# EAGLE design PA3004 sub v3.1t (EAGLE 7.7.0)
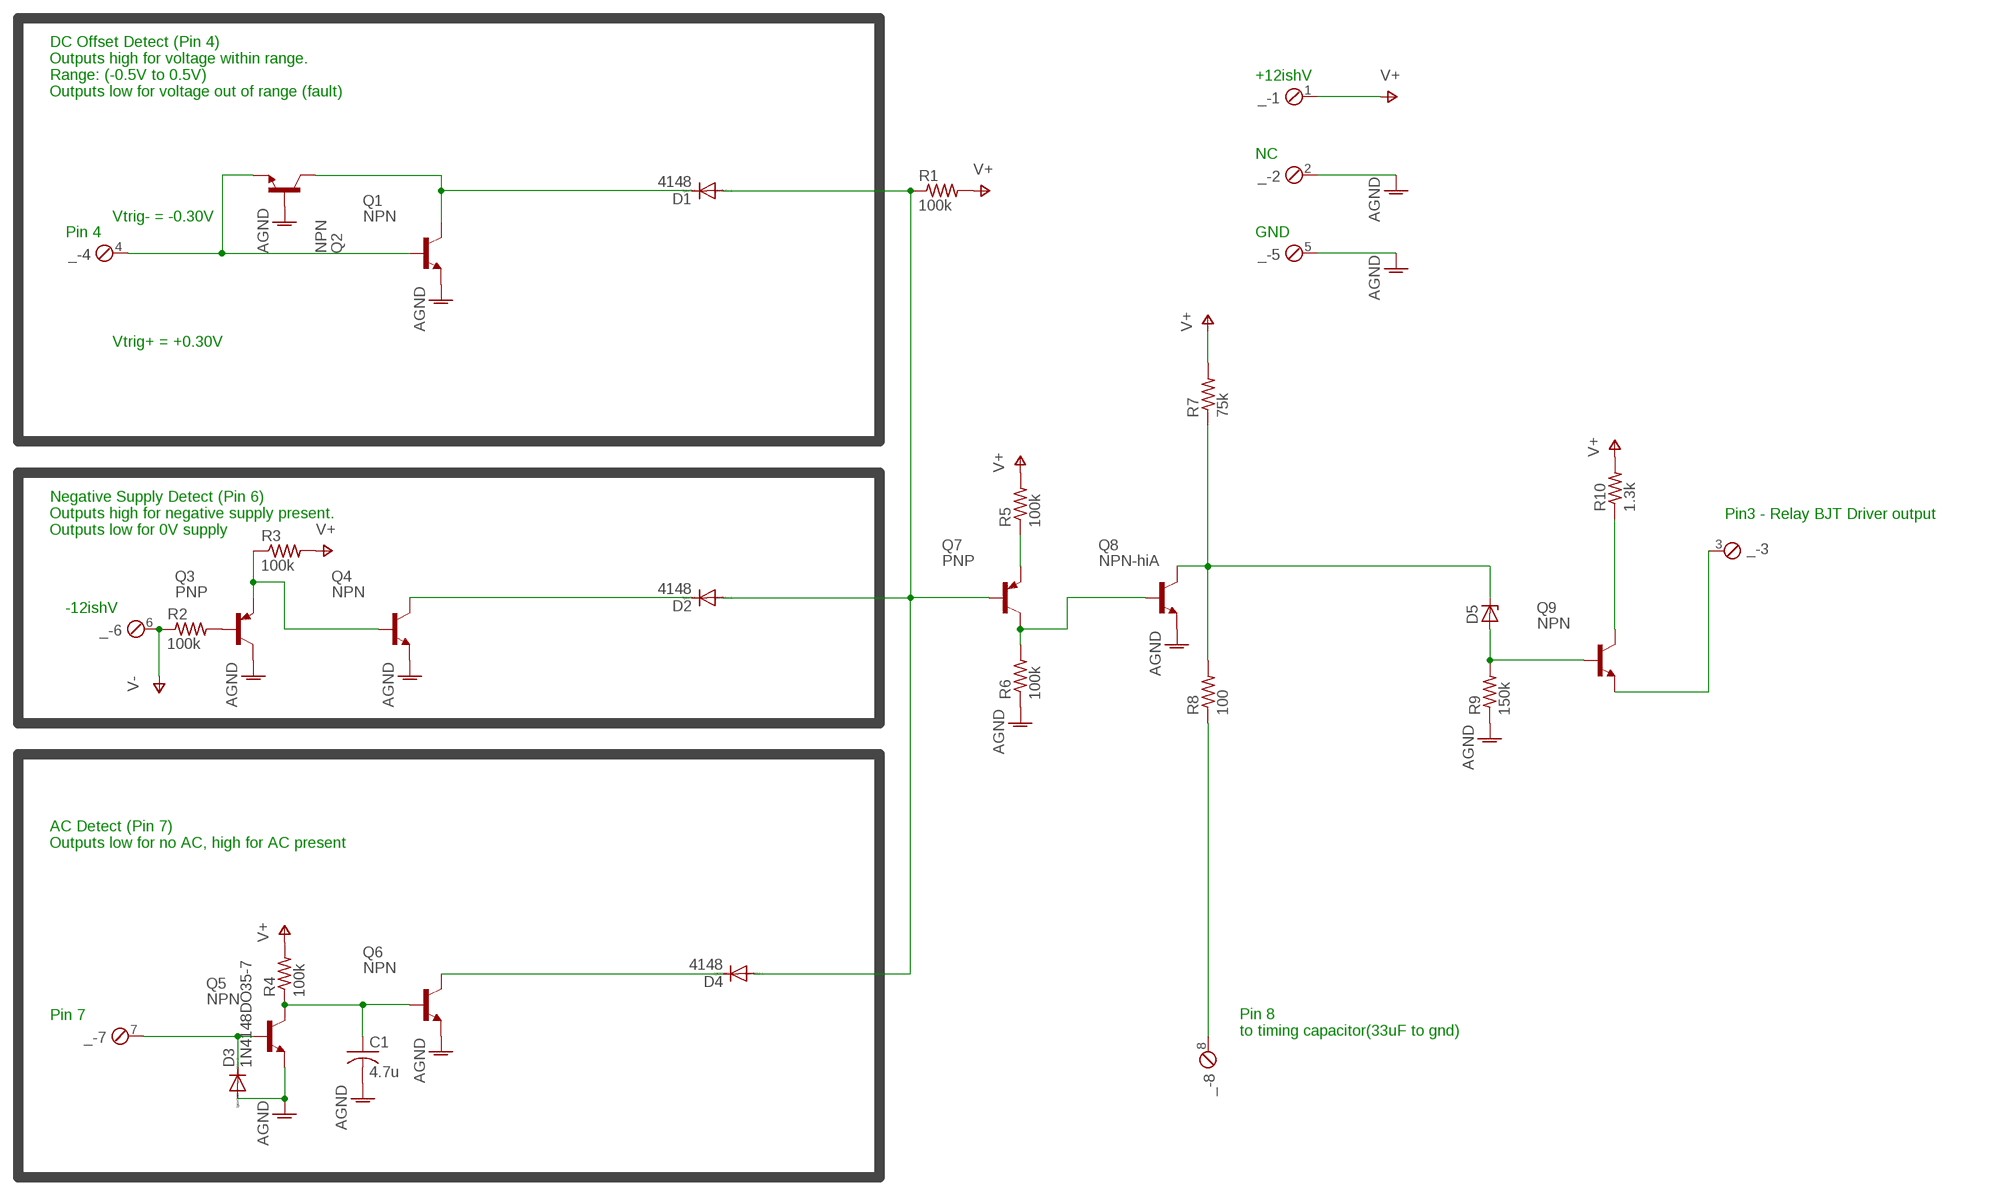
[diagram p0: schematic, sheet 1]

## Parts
_  MPT8  [8POL254]
C1  4.7u  C-US050-024X044  [C050-024X044]
D1  4148  1N4148DO35-7  [DO35-7]
D2  4148  1N4148DO35-7  [DO35-7]
D3  1N4148DO35-7  [DO35-7]
D4  4148  1N4148DO35-7  [DO35-7]
D5  ZENER-DIODEZD-5  [ZDIO-5]
Q1  NPN  KSC1845-THRU  [TO92_BCE]
Q2  NPN  KSC1845-THRU  [TO92_BCE]
Q3  PNP  KSA992-THRU  [TO92_BCE]
Q4  NPN  KSC1845-THRU  [TO92_BCE]
Q5  NPN  KSC1845-THRU  [TO92_BCE]
Q6  NPN  KSC1845-THRU  [TO92_BCE]
Q7  PNP  KSA992-THRU  [TO92_BCE]
Q8  NPN-hiA  KSC1845-THRU  [TO92_BCE]
Q9  NPN  KSC1845-THRU  [TO92_BCE]
R1  100k  R-US_0204/5  [0204/5]
R2  100k  R-US_0204/5  [0204/5]
R3  100k  R-US_0204/5  [0204/5]
R4  100k  R-US_0204/5  [0204/5]
R5  100k  R-US_0204/5  [0204/5]
R6  100k  R-US_0204/5  [0204/5]
R7  75k  R-US_0204/5  [0204/5]
R8  100  R-US_0204/5  [0204/5]
R9  150k  R-US_0204/5  [0204/5]
R10  1.3k  R-US_0204/5  [0204/5]

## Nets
-12V: _.6 R2.1 ; supply symbol labelled V-
AGND: _.2 _.5 C1.2 D3.A Q1.E Q2.B Q3.C Q4.E Q5.E Q6.E Q8.E R6.1 R9.1
N$1: _.4 Q1.B Q2.E
N$2: D1.C Q1.C Q2.C
N$3: D1.A D2.A D4.A Q7.B R1.1
N$4: D4.C Q6.C
N$5: Q3.B R2.2
N$6: Q7.C Q8.B R6.2
N$7: _.7 D3.C Q5.B
N$8: Q7.E R5.1
N$9: C1.1 Q5.C Q6.B R4.1
N$10: Q3.E Q4.B R3.1
N$11: _.8 R8.1
N$12: D5.A Q9.B R9.2
N$13: D5.C Q8.C R7.1 R8.2
N$14: Q9.C R10.1
N$15: D2.C Q4.C
N$16: _.3 Q9.E
V+: _.1 R1.2 R3.2 R4.2 R5.2 R7.2 R10.2

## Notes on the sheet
- +12ishV
- DC Offset Detect (Pin 4)
  Outputs high for voltage within range.
  Range: (-0.5V to 0.5V) 
  Outputs low for voltage out of range (fault)
- NC
- Vtrig- = -0.30V
- Pin 4 | GND
- Vtrig+ = +0.30V
- Pin3 - Relay BJT Driver output
- Negative Supply Detect (Pin 6)
  Outputs high for negative supply present. 
  Outputs low for 0V supply
- -12ishV
- AC Detect (Pin 7)
  Outputs low for no AC, high for AC present
- Pin 7
- Pin 8
  to timing capacitor(33uF to gnd)

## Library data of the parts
_ = con-phoenix-254:MPT8: PHOENIX CONNECTOR; OC_FARNELL: unknown; OC_NEWARK: unknown
C1 = rcl:C-US: CAPACITOR, American symbol
D1-D4 = diode:1N4148: DIODE
D5 = diode:ZENER-DIODE: Z-Diode
Q1 Q2 Q4-Q6 Q8 Q9 = PA3004 Components:KSC1845-THRU
Q3 Q7 = PA3004 Components:KSA992-THRU
R1-R10 = rcl:R-US_: RESISTOR, American symbol

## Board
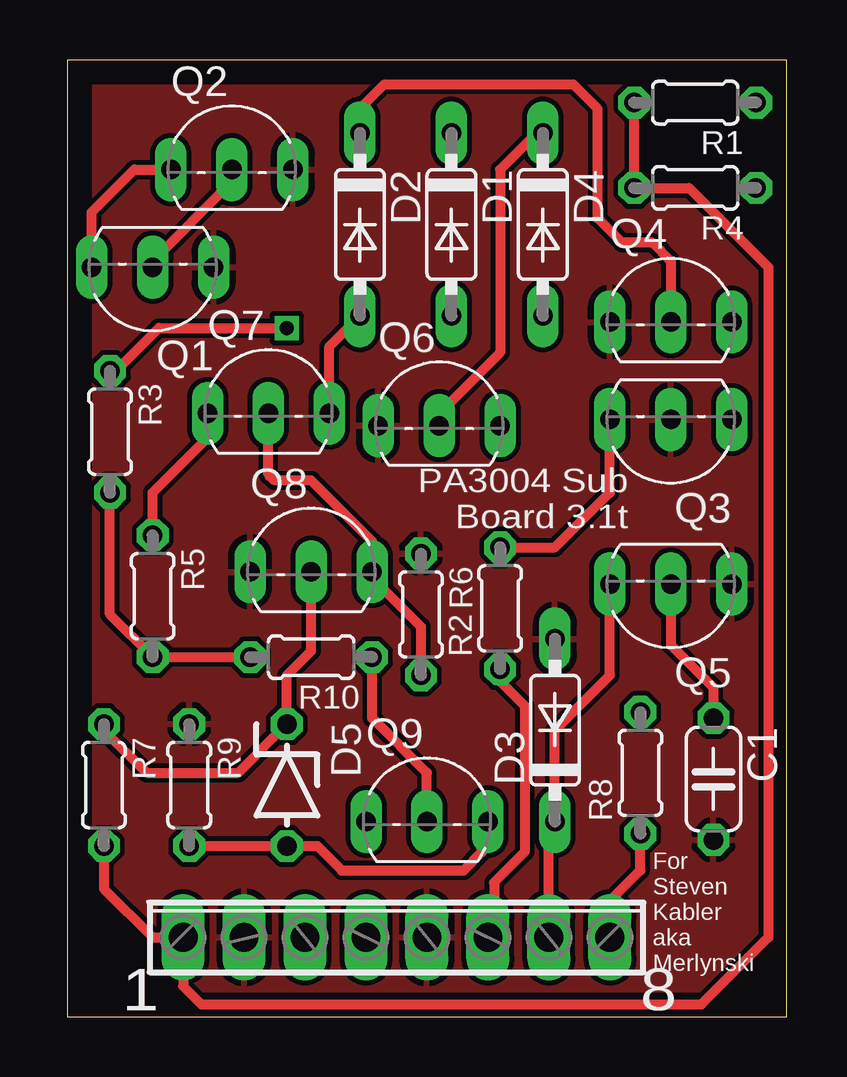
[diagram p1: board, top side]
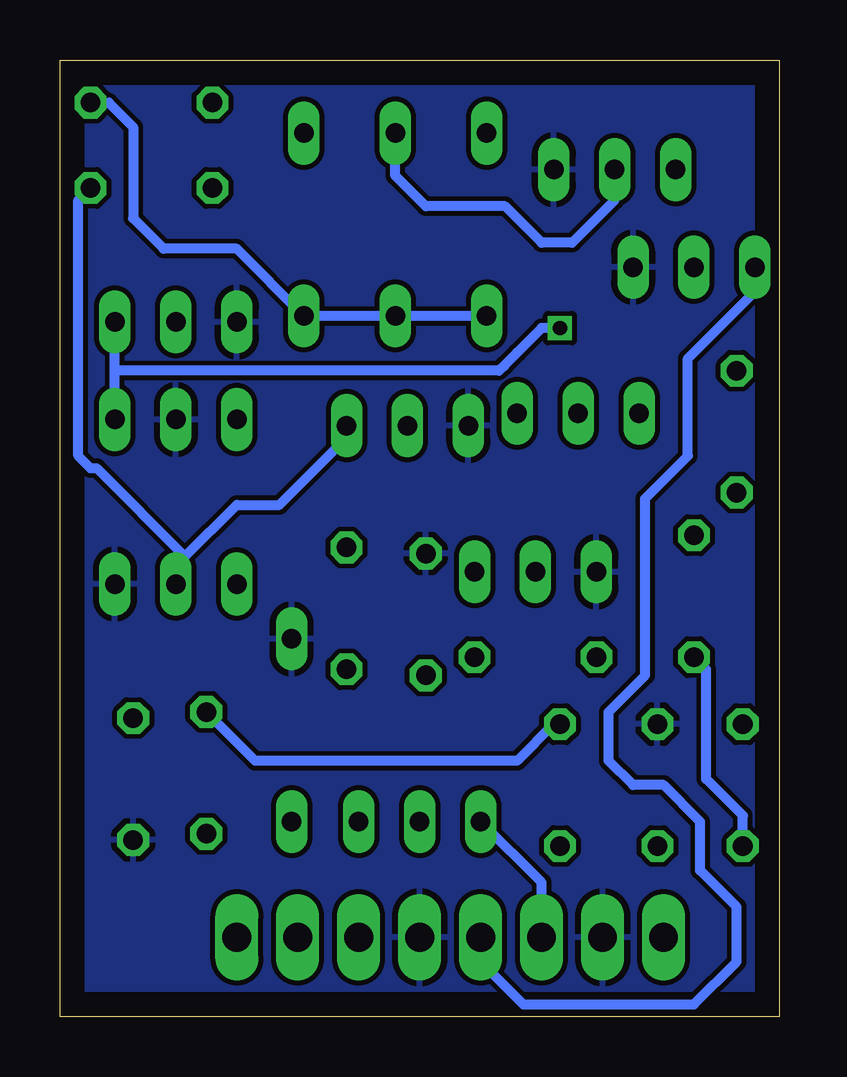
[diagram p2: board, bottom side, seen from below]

Size 29.97 x 39.88 mm. Coordinates in mm from the lower left corner, seen from the top.
Outline: 0,0 29.97,0 29.97,39.88 0,39.88 0,0
Copper layers (1*16): Top 0.035mm / dielectric 1.5mm / Bottom 0.035mm
Design rules "default": minimum track width 10mil, minimum drill 24mil, track to track 8mil, track to pad 8mil, pad to pad 8mil, via to via 8mil, smd to smd 8mil, copper to edge 40mil, drill to drill 8mil, minimum pad ring 10mil, minimum via ring 8mil, stop-mask expansion 4mil, vias tented up to drill 0mil, thermal gap 10mil

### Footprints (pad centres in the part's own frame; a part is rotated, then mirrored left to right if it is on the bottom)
8POL254 = drill 1.2 long: 1 -8.89,0; 2 -6.35,0; 3 -3.81,0; 4 -1.27,0; 5 1.27,0; 6 3.81,0; 7 6.35,0; 8 8.89,0
C050-024X044 = drill 0.813 octagon: 1 -2.54,0; 2 2.54,0
DO35-7 = drill 0.813 long: A 3.81,0; C -3.81,0
ZDIO-5 = drill 0.813 octagon: A 2.54,0; C -2.54,0
TO92_BCE = drill 0.813 long: B 2.54,0; C 0,0; E -2.54,0
0204/5 = drill 0.813 octagon: 1 -2.54,0; 2 2.54,0

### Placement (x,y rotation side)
_  13.72,3.3 0 top
C1  26.92,9.91 270 top
D1  16,33.02 270 top
D2  12.19,33.02 270 top
D3  20.32,11.94 90 top
D4  19.81,33.02 270 top
D5  9.14,9.65 270 top
Q1  3.56,31.24 180 top
Q2  6.86,35.31 0 top
Q3  25.15,24.89 180 top
Q4  25.15,28.96 0 top
Q5  25.15,18.03 180 top
Q6  15.49,24.64 0 top
Q7  8.38,25.15 0 top
Q8  10.16,18.54 0 top
Q9  14.99,8.13 0 top
R1  26.16,38.1 180 top
R2  18.03,17.02 90 top
R3  1.78,24.38 270 top
R4  26.16,34.54 180 top
R5  3.56,17.53 270 top
R6  14.73,16.76 270 top
R7  1.52,9.65 270 top
R8  23.88,10.16 90 top
R9  5.08,9.65 270 top
R10  10.16,14.99 180 top

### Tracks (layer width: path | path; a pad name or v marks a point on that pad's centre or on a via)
-12V
  Top 0.406: R2.1 18.03,13.97 19.05,12.95 19.05,6.86 17.78,5.59 17.78,3.56 _.6
AGND
  pour Top: 0,0 0,39.88 29.97,39.88 29.97,0
  pour Bottom: 0,0 29.97,0 29.97,39.88 0,39.88
N$1
  Top 0.406: Q1.B 1.02,33.53 2.79,35.31 Q2.E
  Bottom 0.406: _.4 12.45,2.29 10.67,0.51 3.56,0.51 1.78,2.29 1.78,4.57 3.3,6.1 3.3,8.13 4.83,9.65 6.1,9.65 7.11,10.67 7.11,12.7 5.59,14.22 5.59,21.59 3.81,23.37 3.81,27.43 1.02,30.23 Q1.B
N$2
  Top 0.406: Q1.C 3.56,31.5 6.86,34.8 Q2.C
  Bottom 0.406: D1.C 16,35.05 14.73,33.78 11.43,33.78 9.91,32.26 8.64,32.26 6.86,34.04 Q2.C
N$3
  Top 0.406: Q7.B 10.92,27.94 D2.A
  Bottom 0.406: D2.A D1.A D4.A 22.61,32 25.65,32 26.92,33.27 26.92,37.08 27.94,38.1 R1.1
N$4
  Top 0.406: D4.C 19.56,36.83 18.03,35.31 18.03,27.69 15.49,25.15 Q6.C
N$5
  Top 0.406: R2.2 20.32,19.56 22.61,21.84 Q3.B
N$6
  Top 0.406: R6.2 14.73,16.26 12.7,18.29 Q8.B 12.7,19.81 10.16,22.35 8.64,22.35 8.38,22.61 Q7.C
N$7
  Top 0.406: _.7 20.07,7.87 D3.C 20.32,11.94 22.61,14.22 Q5.B
N$8
  Top 0.406: R5.1 3.56,21.84 6.1,24.38 6.1,24.89 Q7.E
N$9
  Top 0.406: Q5.C 25.15,15.49 26.92,13.72 C1.1
  Bottom 0.406: Q5.C 25.15,18.8 24.77,19.18 | 24.77,19.18 22.61,21.34 20.83,21.34 18.03,24.13 Q6.B | R4.1 29.21,34.04 29.21,23.37 28.7,22.86 28.45,22.86 24.77,19.18
N$10  (via drill 0.6)
  Top 0.406: R3.1 2.03,26.92 3.81,28.7 v9.14,28.7
  Bottom 0.406: 27.69,26.92 11.68,26.92 11.43,27.18 10.92,27.69 9.91,28.7 v9.14,28.7 | 27.69,26.92 Q4.B | Q3.E 27.69,26.92
N$11
  Top 0.406: _.8 22.61,4.83 23.88,6.1 R8.1
N$12
  Top 0.406: R9.2 D5.A 10.41,7.11 11.43,6.1 16.51,6.1 17.27,6.86 17.27,7.87 Q9.B
N$13
  Top 0.406: R7.1 1.52,11.94 3.3,10.16 7.11,10.16 D5.C 9.14,14.22 10.16,15.24 Q8.C
  Bottom 0.406: R8.2 21.84,10.67 10.92,10.67 9.4,12.19 D5.C
N$14
  Top 0.406: Q9.C 14.99,10.16 12.7,12.45 R10.1
N$15
  Top 0.406: D2.C 12.19,37.85 13.21,38.86 21.08,38.86 22.1,37.85 22.1,33.27 23.11,32.26 24.38,32.26 25.15,31.5 Q4.C
N$16
  Bottom 0.406: _.3 9.91,5.59 Q9.E
V+
  Top 0.406: R7.2 1.52,5.33 3.56,3.3 _.1 4.83,1.27 5.59,0.51 26.42,0.51 29.21,3.3 29.21,31.24 25.91,34.54 R4.2 R1.2 | R3.2 1.78,16.76 R5.2 R10.2
  Bottom 0.406: R7.2 1.52,8.38 3.05,9.91 3.05,14.48 R5.2

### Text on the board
tPlace: PA3004 Sub / Board 3.1t | For / Steven / Kabler / aka / Merlynski | 1 | 8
